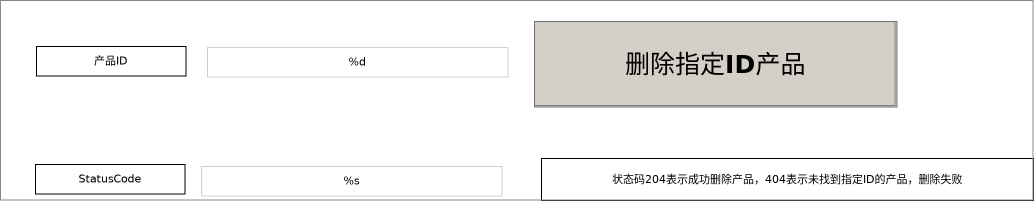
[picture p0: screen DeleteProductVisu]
VISUALIZATION DeleteProductVisu  // 1034x201
    Rectangle (36,46 150x30), "产品ID"
    Textfield (207,47 301x30), "%d", text variable: MAIN.fbDeleteProductById.deleteProductId
        OnMouseDown: write the text variable via Default
    Rectangle (35,164 150x30), "StatusCode"
    Textfield (201,166 301x30), "%s", text variable: MAIN.fbDeleteProductById.nStatusCode
        OnMouseDown: write the text variable via Default
    Rectangle (541,158 493x43), "状态码204表示成功删除产品，404表示未找到指定ID的产品，删除失败"
    Button (534,21 363x86), "删除指定ID产品"
        tap MAIN.fbDeleteProductById.bSend
END_VISUALIZATION
